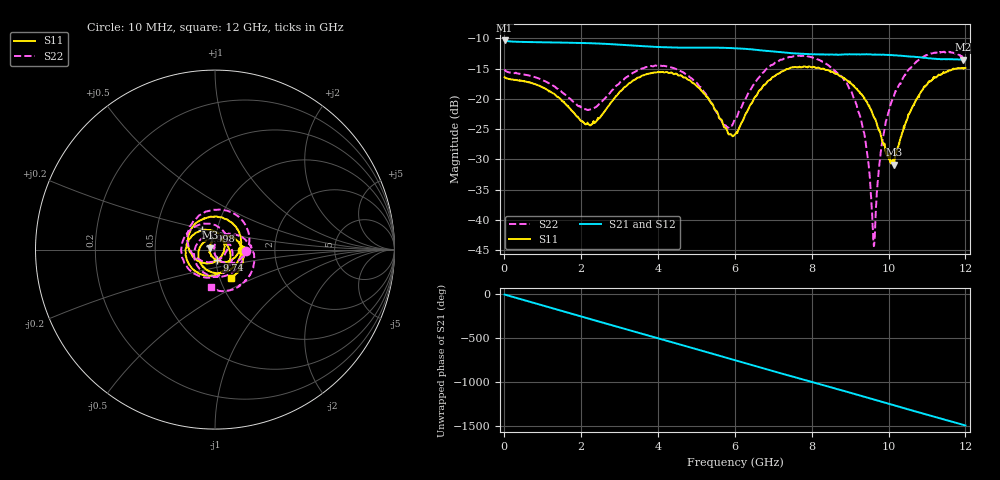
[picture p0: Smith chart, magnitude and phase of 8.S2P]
!Agilent Technologies,E5071C,MY46316741,A.11.02
!Date: Wed Sep 16 11:44:45 2020
!Data & Calibration Information:
!Freq	S11:SOLT2(ON)	S21:SOLT2(ON)	S12:SOLT2(ON)	S22:SOLT2(ON)
!PortZ  Port1:50+j0  Port2:50+j0
!Above PortZ is port z conversion or system Z0 setting when saving the data.
!When reading, reference impedance value at option line is always used.
# Hz S dB R 50
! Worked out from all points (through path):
!   1561 points, 10 MHz to 12 GHz, reference 50 ohm
!   highest |S21| = -10.35 dB at 10 MHz (marker M1); lowest = -13.5 dB at 11.95 GHz (marker M2)
!   group delay of S21, straight-line fit = 344 ps
!   lowest |S11| = -30.9 dB at 10.15 GHz (marker M3), VSWR 1.06, Z = 47.4 + j1.1 ohm
!   |S11| at or under -10 dB: start of sweep to end of sweep
!   |S22| runs from -44.4 to -12.2 dB; largest |S21 - S12| = 0.002
!   S11 on the Smith chart (normalised r, x): 10 MHz: 1.36, -0.01; 4.998 GHz: 0.85, +0.18; 9.74 GHz: 1.01, -0.11; 12 GHz: 1.13, -0.37
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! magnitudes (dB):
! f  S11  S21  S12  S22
! 10 MHz  -16.4  -10.3  -10.4  -15.2
! 1.094 GHz  -18.4  -10.7  -10.7  -17.2
! 2.016 GHz  -23.7  -10.8  -10.8  -21.5
! 2.347 GHz  -24.0  -10.8  -10.8  -21.5
! 3.23 GHz  -17.5  -11.1  -11.1  -16.2
! 4.007 GHz  -15.6  -11.4  -11.4  -14.6
! 4.998 GHz  -17.9  -11.5  -11.5  -17.3
! 5.744 GHz  -24.8  -11.6  -11.6  -24.4
! 6.005 GHz  -25.9  -11.7  -11.7  -23.4
! 6.881 GHz  -17.0  -12.1  -12.1  -14.8
! 8.011 GHz  -14.8  -12.6  -12.6  -13.1
! 8.78 GHz  -16.3  -12.7  -12.7  -16.3
! 9.133 GHz  -18.2  -12.6  -12.6  -20.4
! 9.418 GHz  -20.4  -12.6  -12.6  -27.7
! 9.61 GHz  -22.9  -12.7  -12.7  -43.5
! 9.656 GHz  -23.4  -12.7  -12.7  -40.9
! 9.74 GHz  -25.0  -12.7  -12.7  -32.3
! 10 GHz  -29.7  -12.7  -12.8  -22.2
! 10.15 GHz  -30.9  -12.8  -12.8  -19.4
! 10.89 GHz  -18.4  -13.2  -13.2  -13.1
! 11.95 GHz  -15.0  -13.5  -13.5  -13.1
! 12 GHz  -14.9  -13.5  -13.5  -13.5
